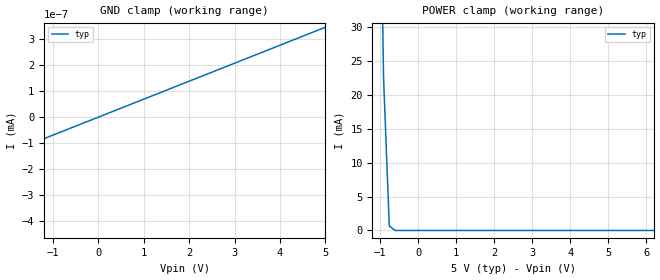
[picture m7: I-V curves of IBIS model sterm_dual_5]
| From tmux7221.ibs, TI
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| sterm_dual_5
[Model]   sterm_dual_5
Model_type   Terminator
|   typ   min   max
C_comp   1.008417e-11   NA   NA
[Voltage Range]   5   NA   NA
[Temperature Range]   27   NA   NA
[Power Clamp Reference]   5   NA   NA
[GND Clamp Reference]   0   NA   NA
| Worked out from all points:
|   GND clamp passes 1 mA (typ) near -5.76 V on its own axis
|   POWER clamp passes 1 mA (typ) near -0.76 V on its own axis
[GND Clamp]
|   Voltage   I(typ)   I(min)   I(max)
-10V      -3.846A    NA         NA
-5.303V   -553.8pA   NA         NA
-5.152V   -360pA     NA         NA
-5V       -347pA     NA         NA
5V        346.8pA    NA         NA
[POWER Clamp]
|   Voltage   I(typ)   I(min)   I(max)
-5V       4.761A     NA         NA
-1.061V   80.13mA    NA         NA
-909.1mV  22.65mA    NA         NA
-757.6mV  658.2uA    NA         NA
-606.1mV  3.286uA    NA         NA
10V       -347pA     NA         NA
